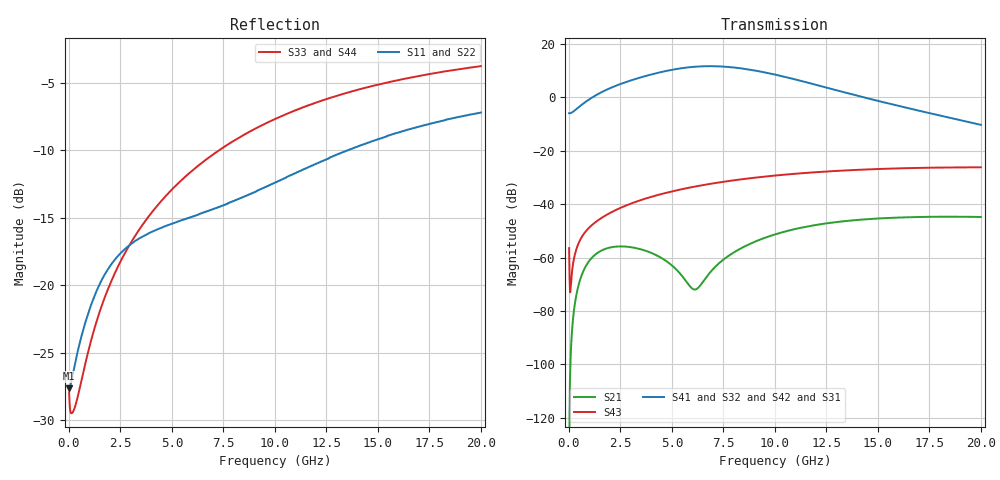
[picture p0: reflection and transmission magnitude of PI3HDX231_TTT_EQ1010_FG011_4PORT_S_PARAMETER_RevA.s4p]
! NPort=4 DATA=2000 NOISE=0 GROUPDELAY=0 COMPLEX_DATAFORMAT=POLAR
! NumOfBlock=1 NumOfParam=0
! .MODEL Smodel S TSTONEFILE=PI3HDX231_TTT_EQ1010_FG011_4PORT_S_PARAMETER_RevA.s4p TYPE=S
!  -- The above .MODEL line can be used for the S element in the netlist.
! The s parameter is extracted from the linear redriver, it is not bi-directional; only s(4,1)s(4,2) and s(3,1)s(3,2)
! should be the insertion loss
!Port definition:
!Port1 = input+
!Port2 = input-
!Port3 = output+
!Port4 = output-
# Hz S MA R  50
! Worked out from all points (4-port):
!   2000 points, 10 MHz to 20 GHz, reference 50 ohm
!   strongest paths, dB at 10 MHz, 5.01 GHz, 10.01 GHz, 15.01 GHz, 20 GHz:
!     S41: -5.9, 10.3, 8.5, -1.3, -10.3
!     S32: -5.9, 10.3, 8.5, -1.3, -10.2
!     S42: -5.9, 10.3, 8.4, -1.5, -10.4
!     S31: -5.9, 10.2, 8.3, -1.7, -10.7
!     S43: -56.5, -35.2, -29.3, -26.9, -26.2
!     S21: -134.8, -63.0, -51.3, -45.4, -44.8
!   lowest |S11| = -27.6 dB at 10 MHz (marker M1), VSWR 1.09, Z = 46 - j0.0776 ohm
!   |S11| at or under -10 dB: start of sweep to 13.55 GHz
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1e7  0.04152 -178.8  1.825e-07 -13.9  0 0.0  0 0.0
     1.825e-07 -14.0  0.04152 -178.8  0 0.0  0 0.0
     0.5042 -0.0  0.5042 180.0  0.04012 -3.2  0.0015 -70.3
     0.5042 180.0  0.5042 -0.0  0.0015 -70.3  0.04012 -3.2
4.25e9  0.1606 -140.8  0.001101 -6.9  2.361e-10 -149.9  1.566e-10 -134.1
        0.001103 -6.9  0.1606 -140.9  1.519e-10 -134.4  2.443e-10 -149.5
        2.811 -43.6  2.816 136.1  0.1953 -100.1  0.01462 65.5
        2.833 136.1  2.828 -42.9  0.01459 65.4  0.1954 -100.1
6.19e9  0.1816 -137.8  0.000253 52.7  2.311e-09 147.8  1.314e-09 -174.9
        0.0002563 51.7  0.1814 -138.0  1.27e-09 -174.3  2.407e-09 147.4
        3.717 -104.0  3.732 75.8  0.2733 -105.9  0.02165 54.8
        3.755 75.6  3.747 -103.2  0.02158 54.7  0.2734 -105.9
8.13e9  0.2069 -133.2  0.00134 99.7  1.073e-08 87.8  7.31e-09 135.9
        0.001332 99.2  0.2062 -133.4  7.118e-09 137.4  1.116e-08 86.5
        3.518 -168.5  3.555 11.3  0.3468 -111.0  0.02846 42.7
        3.574 10.9  3.554 -167.6  0.02834 42.8  0.3469 -111.0
1.066e10  0.2532 -128.8  0.003209 77.8  4.053e-08 19.6  3.276e-08 61.6
          0.00319 77.5  0.2518 -129.0  3.236e-08 63.5  4.157e-08 17.5
          2.267 117.8  2.321 -62.6  0.433 -117.2  0.03628 26.3
          2.326 -63.2  2.296 118.9  0.03616 26.4  0.4331 -117.2
1.364e10  0.3178 -128.4  0.004941 47.0  1.131e-07 -47.5  9.184e-08 -16.1
          0.004908 46.7  0.3158 -128.4  9.21e-08 -14.3  1.142e-07 -49.7
          1.122 52.9  1.169 -128.5  0.5192 -123.8  0.04322 6.7
          1.165 -129.3  1.142 54.2  0.04315 7.0  0.5191 -123.8
2e10  0.4355 -135.6  0.005793 -4.2  3.741e-07 -160.9  2.789e-07 -140.6
      0.005747 -4.3  0.4338 -135.4  2.835e-07 -139.6  3.712e-07 -162.6
      0.2924 -46.7  0.309 128.0  0.6464 -135.0  0.04884 -32.3
      0.3049 127.6  0.3012 -45.3  0.04894 -32.1  0.6461 -135.0
